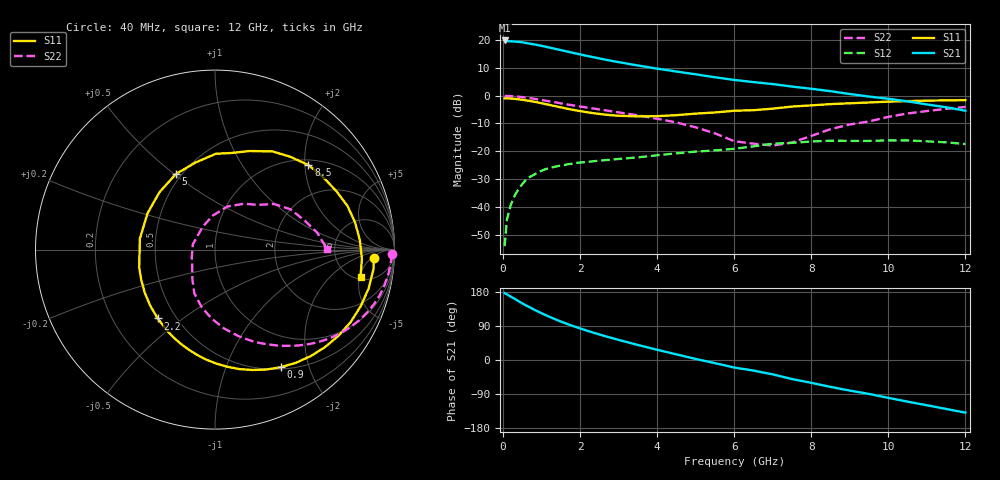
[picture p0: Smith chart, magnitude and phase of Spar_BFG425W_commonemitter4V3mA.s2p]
! Filename: 43bfg425.001
! BFG425W Field C1
! V1=8.107E-001V,V2=4.000E+000V, I1=2.873E-005A, I2=3.000E-003A
# GHz  S  MA  R 50
!  S11  S21  S12  S22
!Freq(GHz)  Mag  Ang  Mag  Ang  Mag  Ang  Mag  Ang
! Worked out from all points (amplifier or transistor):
!   44 points, 40 MHz to 12 GHz, reference 50 ohm
!   highest |S21| = 19.7 dB at 40 MHz (marker M1)
!   |S21| within 3 dB of that: start of sweep to 1.35 GHz
!   unconditionally stable (mu >= 1): 2.855 GHz to end of sweep
!   at 700 MHz: K = 0.25, MSG = 23.8 dB, |S12| = -29.1 dB
!   at 2.4 GHz: K = 0.84, MSG = 18.5 dB, |S12| = -23.5 dB
!   at 12 GHz: K = 1.64, MAG = 1.3 dB, |S12| = -17.4 dB
!   S11 on the Smith chart (normalised r, x): 40 MHz: 14, -6; 900 MHz: 0.53, -1.58; 2.2 GHz: 0.40, -0.41; 5 GHz: 0.47, +0.51; 8.5 GHz: 1.12, +2.09; 12 GHz: 5.39, -5.16
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0.04  0.885 -3.1  9.697 176.6  0.002 54.7  0.984 -1.6
0.1  0.89 -7.1  9.446 173.3  0.006 77.5  0.983 -3.9
0.2  0.883 -14.1  9.355 167.2  0.011 76.3  0.976 -7.9
0.3  0.871 -21.2  9.261 161.6  0.016 73.6  0.966 -11.7
0.5  0.839 -34.9  8.988 149.3  0.026 66.3  0.936 -19.1
0.7  0.798 -48.0  8.479 138.6  0.035 59.0  0.897 -25.8
0.9  0.751 -60.6  8.02 128.3  0.042 52.6  0.853 -32.0
1.2  0.68 -78.3  7.237 114.1  0.05 44.1  0.787 -40.1
1.6  0.593 -100.2  6.289 97.6  0.057 35.4  0.706 -49.2
1.9  0.541 -115.3  5.648 86.7  0.062 30.3  0.653 -55.2
2.2  0.499 -129.8  5.093 76.7  0.065 26.4  0.605 -60.8
2.6  0.459 -148.6  4.471 64.4  0.069 22.2  0.55 -67.9
3  0.434 -166.7  3.964 53.0  0.073 18.8  0.499 -74.9
3.5  0.423 171.7  3.452 39.7  0.078 15.1  0.441 -83.7
4.5  0.445 134.0  2.692 14.9  0.092 6.8  0.329 -103.1
5  0.474 117.4  2.398 2.8  0.099 0.8  0.269 -115.4
6  0.534 89.4  1.903 -19.9  0.111 -11.0  0.152 -146.8
6.5  0.546 80.3  1.74 -27.9  0.123 -10.4  0.137 -161.1
7.5  0.634 59.6  1.446 -50.3  0.142 -28.7  0.144 118.7
8.5  0.702 42.1  1.195 -71.0  0.155 -45.2  0.25 73.9
10.5  0.795 11.0  0.786 -109.9  0.157 -80.6  0.477 28.1
12  0.825 -10.7  0.535 -138.8  0.135 -112.2  0.625 0.1
